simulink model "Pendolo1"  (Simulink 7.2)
settings: Solver=ode45  StartTime=0.0  StopTime=10  RelTol=1e-3
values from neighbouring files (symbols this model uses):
  Cm = 1    [PendParams.m]
  g = 9.81*m/s^2    (= 9.81)    [motoreDC0.m]    (also in PendParams.m = 9.806)
  l = 1.2    [PendParams.m]
  M = 0.25    [PendParams.m]
  q0 = pi/2    (= 1.57079632679)    [PendParams.m]
  w0 = 0    [PendParams.m]
libraries: simulink x1

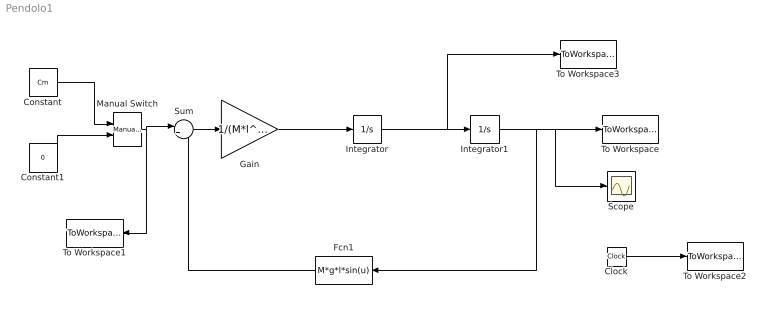
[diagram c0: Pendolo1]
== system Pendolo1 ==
  Clock : Clock
  Constant : Constant  Value=Cm  OutDataType=sfix(16)  OutScaling=2^0
  Constant1 : Constant  Value=0  OutDataType=sfix(16)  OutScaling=2^0
  Fcn1 : Fcn  Orientation=left  Expr=M*g*l*sin(u)
  Gain : Gain  Gain=1/(M*l^2)  ParameterDataType=sfix(16)  ParameterScaling=2^0  OutDataType=sfix(16)  OutScaling=2^0
  Integrator : Integrator  InitialCondition=w0
  Integrator1 : Integrator  InitialCondition=q0
  Manual Switch : simulink/Signal Routing/Manual Switch  SystemSampleTime=-1  sw=0  action=0  varsize=off
  Scope : Scope
  Sum : Sum  Inputs=|+-  OutDataType=sfix(16)  OutScaling=2^0
  To Workspace : ToWorkspace  VariableName=q  SampleTime=-1  SaveFormat=Array
  To Workspace1 : ToWorkspace  VariableName=Ci  SampleTime=-1  SaveFormat=Array
  To Workspace2 : ToWorkspace  VariableName=t  SampleTime=-1  SaveFormat=Array
  To Workspace3 : ToWorkspace  VariableName=w  SampleTime=-1  SaveFormat=Array
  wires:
  Gain/1 -> Integrator/1
  Manual Switch/1 -> Sum/1, To Workspace1/1
  Constant1/1 -> Manual Switch/2
  Clock/1 -> To Workspace2/1
  Constant/1 -> Manual Switch/1
  Integrator/1 -> Integrator1/1, To Workspace3/1
  Integrator1/1 -> To Workspace/1, Scope/1, Fcn1/1
  Fcn1/1 -> Sum/2
  Sum/1 -> Gain/1
